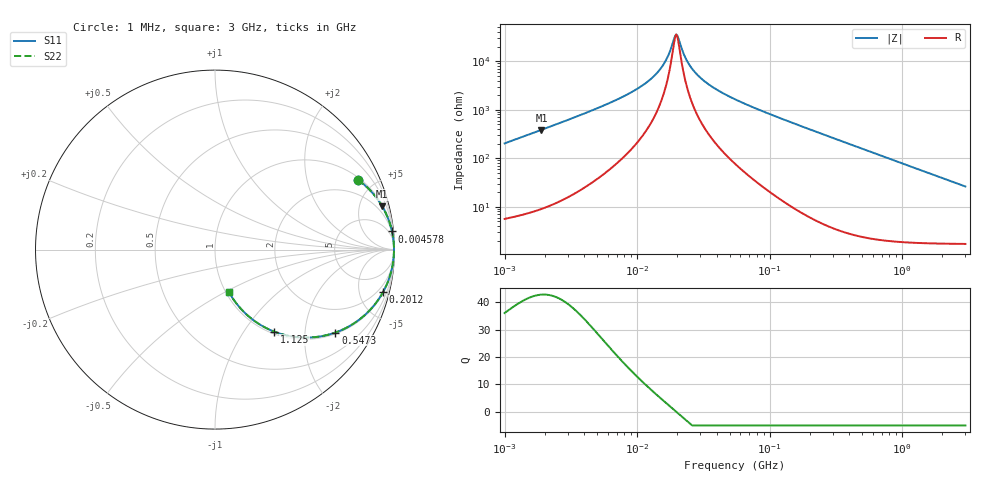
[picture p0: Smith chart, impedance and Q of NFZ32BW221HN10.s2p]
! NFZ32BW221HN10
# Hz S RI R 50
!Freq.(Hz) S11(Real) S11(Imag) S21(Real) S21(Imag) S12(Real) S12(Imag) S22(Real) S22(Imag)
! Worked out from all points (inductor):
!   401 points, 1 MHz to 3 GHz, reference 50 ohm
!   read as one part in series: L = 32.1 uH near 1.041 MHz
!   highest Q = 42.8 at 1.897 MHz (marker M1), where L = 32.3 uH
!   self-resonance near 19.73 MHz
!   S11 on the Smith chart (normalised r, x): 1 MHz: 1.11, +4.05; 4.578 MHz: 2, +19; 201.2 MHz: 1.12, -7.87; 547.3 MHz: 1.05, -2.87; 1.125 GHz: 1.04, -1.39; 3 GHz: 1.03, -0.52
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1000000  0.7978 0.388  0.2022 -0.388  0.2022 -0.388  0.7978 0.388
1897447  0.9321 0.2402  0.0679 -0.2402  0.0679 -0.2402  0.9321 0.2402
3823119  0.9811 0.1224  0.0189 -0.1224  0.0189 -0.1224  0.9811 0.1224
4577760  0.9863 0.1011  0.0137 -0.1011  0.0137 -0.1011  0.9863 0.1011
9600343  0.9956 0.0393  0.00444 -0.0393  0.00444 -0.0393  0.9956 0.0393
1.461624e7  0.9969 0.0153  0.00305 -0.0153  0.00305 -0.0153  0.9969 0.0153
1.648134e7  0.9971 0.00913  0.00289 -0.00913  0.00289 -0.00913  0.9971 0.00913
1.896016e7  0.9972 0.00206  0.0028 -0.00206  0.0028 -0.00206  0.9972 0.00206
1.973457e7  0.9972 5.43e-05  0.00279 -5.43e-05  0.00279 -5.43e-05  0.9972 5.43e-05
2.054061e7  0.9972 -0.00195  0.0028 0.00195  0.0028 0.00195  0.9972 -0.00195
2.41077e7  0.9971 -0.01  0.00289 0.01  0.00289 0.01  0.9971 -0.01
2.829425e7  0.9969 -0.0184  0.00313 0.0184  0.00313 0.0184  0.9969 -0.0184
3.670325e7  0.9961 -0.033  0.00389 0.033  0.00389 0.033  0.9961 -0.033
5.477226e7  0.9935 -0.0602  0.00648 0.0602  0.00648 0.0602  0.9935 -0.0602
2.011837e8  0.9362 -0.2369  0.0638 0.2369  0.0638 0.2369  0.9362 -0.2369
2.094008e8  0.9314 -0.2454  0.0686 0.2454  0.0686 0.2454  0.9314 -0.2454
3.453811e8  0.8351 -0.3643  0.1649 0.3643  0.1649 0.3643  0.8351 -0.3643
5.473095e8  0.6706 -0.4622  0.3294 0.4622  0.3294 0.4622  0.6706 -0.4622
8.005644e8  0.4903 -0.49  0.5097 0.49  0.5097 0.49  0.4903 -0.49
1.125055e9  0.3315 -0.4578  0.6685 0.4578  0.6685 0.4578  0.3315 -0.4578
1.818868e9  0.1669 -0.3531  0.8331 0.3531  0.8331 0.3531  0.1669 -0.3531
3e9  0.0778 -0.237  0.9222 0.237  0.9222 0.237  0.0778 -0.237
